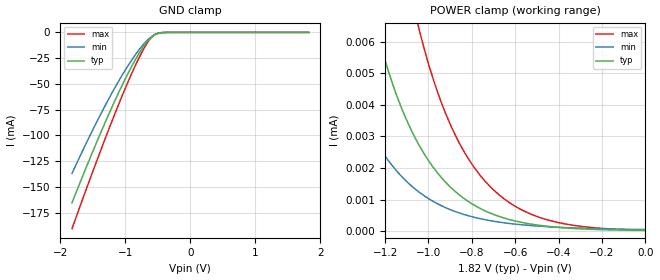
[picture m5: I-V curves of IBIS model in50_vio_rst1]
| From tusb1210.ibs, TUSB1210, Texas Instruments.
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|   Model: in50_vio_rst1
|   Description:  Input buf under VIO (Output High in RESET mode)
[Model]   in50_vio_rst1
Model_type   Input
Polarity   Non-Inverting
Vinh =   1.014
Vinl =   0.815
|variable   typ   min   max
C_comp   1.448p   0.995p   2.116p
[Model Spec]
|Thresholds   typ   min   max
Vinh+   1.014   0.958   1.069
Vinh-   0.993   0.939   1.048
Vinl+   0.835   0.789   0.881
Vinl-   0.815   0.770   0.860
[Temperature Range]   27   125   -40
[Voltage Range]   1.82   1.72   1.92
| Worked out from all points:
|   GND clamp passes 1 mA (typ) near -0.50 V on its own axis
[GND Clamp]
| in50_vio_rst1
|Voltage   I(typ)   I(min)   I(max)
-1.82V    -165.4mA   -136.8mA   -190.4mA
-1.575V   -126.9mA   -104.1mA   -147.7mA
-1.37V    -96.14mA   -78.35mA   -113.1mA
-1.166V   -67mA      -54.31mA   -79.8mA
-1.002V   -45.29mA   -36.69mA   -54.5mA
-838.4mV  -25.69mA   -21.04mA   -31.13mA
-715.7mV  -13.21mA   -11.19mA   -15.83mA
-633.9mV  -6.661mA   -6.022mA   -7.625mA
-552.1mV  -2.345mA   -2.477mA   -2.317mA
-470.3mV  -502.1uA   -715.6uA   -375.2uA
-347.6mV  -20.61uA   -62.98uA   -7.086uA
1.82V     20.44nA    59.47nA    16.09nA
[POWER Clamp]
| in50_vio_rst1
|Voltage   I(typ)   I(min)   I(max)
-1.82V    55.9uA     26.14uA    111.3uA
-1.452V   14.97uA    6.638uA    32.13uA
-1.329V   9.23uA     4.057uA    20.36uA
-1.247V   6.598uA    2.899uA    14.83uA
-1.145V   4.27uA     1.893uA    9.82uA
-1.043V   2.716uA    1.232uA    6.385uA
-961.1mV  1.867uA    875.6nA    4.463uA
-879.3mV  1.27uA     626nA      3.08uA
-797.5mV  855.7nA    452.2nA    2.098uA
-695.3mV  516nA      307.6nA    1.274uA
-429.4mV  135.1nA    131nA      315.4nA
0V        20.44nA    50.05nA    27.66nA
